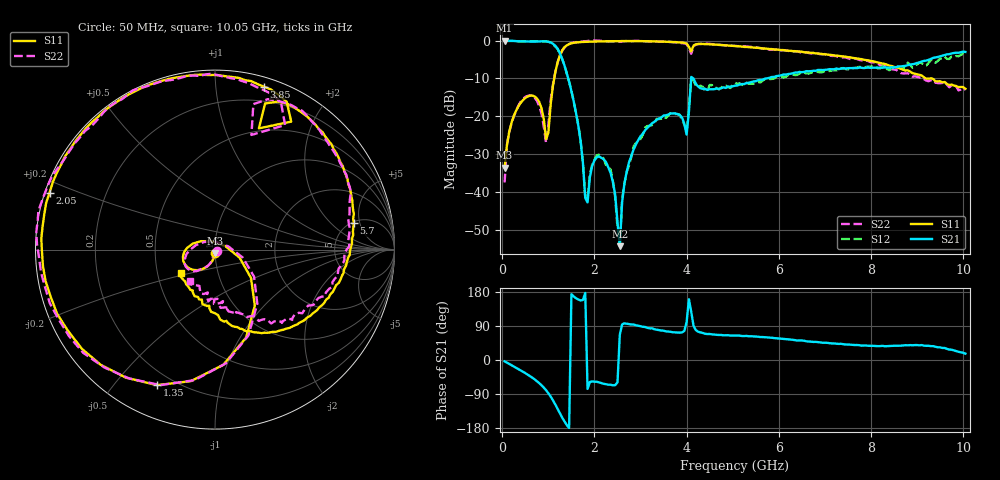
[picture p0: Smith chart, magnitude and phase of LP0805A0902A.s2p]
! AVX THIN FILM OPERATION
! 0805 Size Low Pass Filter P/N  LP0805A0902AWTR
! Network Analyzer HP8720ES.07.64: Feb 23, 2000 Serial No. US39172382
! Hewlett-Packard
!  2 Feb 2003  02:33:11
! Frequency  S11  S21  S12  S22
# HZ  S  DB R  50
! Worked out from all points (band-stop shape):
!   201 points, 50 MHz to 10.05 GHz, reference 50 ohm
!   highest |S21| = 0.00 dB at 50 MHz (marker M1); lowest = -54.4 dB at 2.55 GHz (marker M2)
!   |S21| within 3 dB of the highest: start of sweep to 1.235 GHz; 9.969 GHz to end of sweep
!   lowest |S11| = -33.6 dB at 50 MHz (marker M3), VSWR 1.04, Z = 50.1 - j2.08 ohm
!   |S11| at or under -10 dB: start of sweep to 1.126 GHz; 9.196 GHz to 9.28 GHz (84.31 MHz wide, 0.913 % of centre); 9.312 GHz to end of sweep
!   |S22| runs from -37.5 to 0.1 dB; largest |S21 - S12| = 0.15
!   S11 on the Smith chart (normalised r, x): 50 MHz: 1.00, -0.04; 1.35 GHz: 0.14, -0.65; 2.05 GHz: 0.01, +0.17; 3.85 GHz: 0.07, +1.34; 5.7 GHz: 5.16, +4.06; 10.05 GHz: 0.66, -0.18
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5e7  -33.63 -86.4  -0.00 -3.6  -0.00 -3.5  -37.54 -32.7
1.5e8  -24.15 -102.8  -0.07 -10.3  -0.07 -9.9  -24.16 -104.2
4.5e8  -15.71 -136.2  -0.18 -30.8  -0.16 -30.9  -15.41 -134.9
9.5e8  -26.11 110.1  -0.19 -79.8  -0.18 -79.6  -27.04 88.1
1.15e9  -8.34 -54.6  -1.33 -117.4  -1.56 -116.6  -8.33 -52.0
1.35e9  -1.71 -113.2  -6.61 -162.1  -6.49 -162.9  -1.79 -111.9
1.75e9  -0.33 -174.4  -32.36 158.5  -32.70 157.0  -0.20 -172.5
1.85e9  -0.27 176.4  -42.84 -76.2  -41.99 -80.1  -0.07 178.5
2.05e9  -0.22 161.0  -30.92 -57.4  -30.35 -57.8  0.02 164.5
2.35e9  -0.13 142.1  -35.02 -65.2  -34.10 -65.7  -0.18 146.2
2.55e9  -0.12 131.3  -54.41 66.6  -54.07 77.7  -0.24 134.7
2.65e9  -0.10 126.1  -37.83 96.8  -37.82 90.5  -0.13 128.9
2.85e9  -0.11 116.5  -28.79 93.7  -27.96 92.8  -0.08 119.2
3.4e9  -0.24 92.4  -20.62 78.9  -20.76 73.9  -0.25 95.2
3.85e9  -0.46 73.2  -19.64 72.2  -19.65 70.2  -0.58 75.8
4e9  -0.77 64.1  -24.85 100.0  -24.09 101.4  -0.92 65.9
4.1e9  -2.87 70.1  -9.59 127.2  -10.25 122.5  -3.48 72.4
5.05e9  -1.41 33.2  -11.91 64.5  -11.13 61.4  -1.39 36.1
5.7e9  -2.07 10.9  -10.07 60.1  -10.21 56.3  -2.15 16.1
6.75e9  -3.25 -22.9  -7.96 47.7  -8.30 46.5  -3.27 -17.1
8.4e9  -6.61 -71.2  -7.16 36.7  -7.82 30.2  -7.43 -60.3
1.005e10  -12.73 -145.1  -2.98 16.7  -3.91 11.4  -13.03 -128.6
